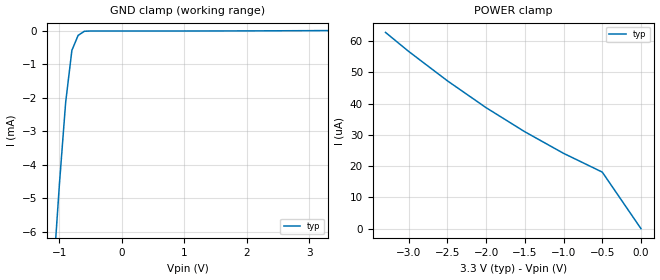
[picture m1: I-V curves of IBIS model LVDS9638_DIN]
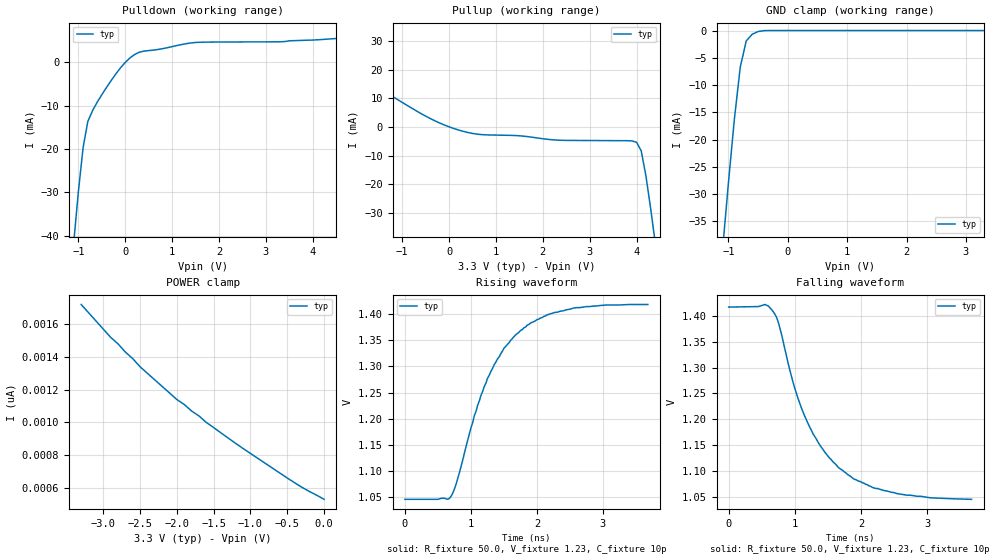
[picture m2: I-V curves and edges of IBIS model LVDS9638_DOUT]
|   Texas Instruments Incorporated
|   Data Transmissions Products
|   IBIS Model for SN65LVDS9638
|   8D SOIC Package
[IBIS Ver]   2.1
[Comment char]   |_char
[File name]   lvds9638.ibs
[File Rev]   2.0
[Date]   27May98
[Source]   File originated at Texas Instruments Incorporated.
   Data Transmission Products Group. All data based on
   Bench Measurements.
[Notes]   Model revved in Nov02 to fix common-mode bug  -TMF-
[Disclaimer]
(C) Copyright Texas Instruments Incorporated 1997
   All rights reserved
  Texas Instruments Incorporated hereby grants the user of this IBIS
model a non-exclusive, nontransferable license to use this IBIS model
under the following terms.  Before using this IBIS model, the user
should read this license.  If the user does not accept these terms,
the IBIS model should be returned to Texas Instruments within 30 days.
  The user is granted this license only to use the IBIS model and
is not granted rights to sell, load, rent, lease or license the IBIS
model in whole or in part, or in modified form to anyone other than
user.  User may modify the IBIS model to suit its specific applications
but rights to derivative works and such modifications shall belong to
Texas Instruments.
  This IBIS model is provided on an "AS IS" basis and Texas Instruments
makes absolutely no warranty with respect to the information contained
herein.  TEXAS INSTRUMENTS DISCLAIMS AND CUSTOMER WAIVES ALL WARRANTIES,
EXPRESS OR IMPLIED, INCLUDING WARRANTIES OF MERCHANTABILITY OR FITNESS
FOR A PARTICULAR PURPOSE. The entire risk as to quality and performance
is with the Customer. ACCORDINGLY, IN NO EVENT SHALL THE COMPANY BE LIABLE
FOR ANY DAMAGES, WHETHER IN CONTRACT OR TORT,INCLUDING ANY LOST PROFITS
OR OTHER INCIDENTAL, CONSEQUENTIAL, EXEMPLARY, OR PUNITIVE DAMAGES ARISING
OUT OF THE USE OR APPLICATION OF THE IBIS model provided in this package.
Further, Texas Instruments reserves the right to discontinue or make changes
without notice to any product herein to improve reliability, function, or
design. Texas Instruments does not convey any license under patent rights
or any other intellectual property rights, including those of third parties.
Contact Texas Instruments at ATTN:DATA TRANSMISSIONS
[Copyright]   Copyright 1997, Texas Instruments, All Rights Reserved
[Component]   SN65LVDS9638D
[Manufacturer]  Texas Instruments Incorporated
[Package]
|   typ   min   max
R_pkg   0.036   0.033   0.039
L_pkg   3.340nH   2.445nH   4.233nH
C_pkg   0.470pF   0.308pF   0.631pF
[Pin]   signal_name   model_name   R_pin   L_pin   C_pin
1   VCC   POWER   0.034   4.233n   0.630p
2   1A   LVDS9638_DIN   0.038   2.445n   0.309p
3   2A   LVDS9638_DIN   0.039   2.448n   0.309p
4   GND   GND   0.033   4.231n   0.631p
5   2Z   LVDS9638_DOUT   0.033   4.230n   0.630p
6   2Y   LVDS9638_DOUT   0.039   2.450n   0.308p
7   1Z   LVDS9638_DOUT   0.039   2.448n   0.309p
8   1Y   LVDS9638_DOUT   0.033   4.231n   0.630p
[Diff_pin]   inv_pin   vdiff   tdelay_typ   tdelay_min   tdelay_max
| The 'xY' pin is Diff_pin and the 'xZ' pin is the inv_pin
6   5   NA   0 0 0
8   7   NA   0 0 0
| Models and submodels in the file (2): LVDS9638_DIN (Input), LVDS9638_DOUT (3-state)
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|   Driver Input  MODEL
[Model]   LVDS9638_DIN
Model_type   Input
|Signals   1A,2A
Vinh = 2.0
Vinl = 0.8
|   typ   min   max
C_comp   1.0pF   NA   NA
|   typ   min   max
[Temperature Range]   25.0   NA   NA
[Voltage range]   3.3V   3.0V   3.6V
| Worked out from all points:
|   GND clamp passes 1 mA (typ) near -0.83 V on its own axis
[GND_clamp]
|   Voltage   I(typ)   I(min)   I(max)
-3.3V     -81mA      NA         NA
-1.1V     -7.36mA    NA         NA
-1V       -4.59mA    NA         NA
-900mV    -2.14mA    NA         NA
-800mV    -579uA     NA         NA
-700mV    -131uA     NA         NA
-600mV    -7.97uA    NA         NA
3.3V      12.9uA     NA         NA
[Power_clamp]
| Note that the[POWER_clamp]voltage table is referenced to Vcc
| and is calculated using Vtable=Vcc - Vmeasured.
|   Voltage   I(typ)   I(min)   I(max)
-3.3V     62.8uA     NA         NA
-3V       56.7uA     NA         NA
-2.5V     47.3uA     NA         NA
-2V       38.7uA     NA         NA
-1.5V     31uA       NA         NA
-1V       24.1uA     NA         NA
-500mV    18.1uA     NA         NA
0V        0A         NA         NA
|   Driver Output  MODEL
[Model]   LVDS9638_DOUT
Model_type   3-state
| Signals   1Y,1Z,2Y,2Z
Vmeas = 1.2V   |Reference voltage for timing measurements
Cref = 10pF   |Timing specification test load capacitance value
Rref = 50   |Note: 50 Ohm load; single ended configuration
Vref = 1.23V   |Timing specification test load voltage
| variable   typ   min   max
C_comp   1.0pF   NA   NA
|   typ   min   max
[Temperature Range]   25.0   NA   NA
[Voltage range]   3.3V   3.0V   3.6V
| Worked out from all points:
|   slope of the pulldown table from 0 to 0.495 V, typ, clamps not added: 182 ohm
|   slope of the pullup table from 0 to 0.495 V, typ, clamps not added: 216 ohm
|   GND clamp passes 1 mA (typ) near -0.63 V on its own axis
|   rising waveform, R_fixture 50.0, V_fixture 1.23, C_fixture 10p: 20-80 % time 692ps typ, NA min, NA max; typ from 1.04 V to 1.42 V
|   falling waveform, R_fixture 50.0, V_fixture 1.23, C_fixture 10p: 20-80 % time 728ps typ, NA min, NA max; typ from 1.42 V to 1.04 V
[Pulldown]
|   Voltage   I(typ)   I(min)   I(max)
-3.3V     -343mA     NA         NA
-1.1V     -41.6mA    NA         NA
-1V       -29.8mA    NA         NA
-900mV    -19.7mA    NA         NA
-800mV    -13.7mA    NA         NA
-600mV    -9.24mA    NA         NA
-200mV    -2.67mA    NA         NA
100mV     992uA      NA         NA
300mV     2.32mA     NA         NA
1.5V      4.56mA     NA         NA
4V        5.12mA     NA         NA
6.6V      7.6mA      NA         NA
[Pullup]
|   Voltage   I(typ)   I(min)   I(max)
| Note that the[Pullup]voltage table is referenced to Vcc
| and is calculated using Vtable=Vcc - Vmeasured.
-3.3V     35mA       NA         NA
-1.2V     10.6mA     NA         NA
-500mV    3.81mA     NA         NA
100mV     -516uA     NA         NA
700mV     -2.67mA    NA         NA
2.3V      -4.58mA    NA         NA
4V        -5.33mA    NA         NA
4.1V      -8.38mA    NA         NA
4.2V      -17.1mA    NA         NA
4.3V      -28.4mA    NA         NA
4.4V      -40.7mA    NA         NA
6.6V      -343mA     NA         NA
[GND_clamp]
|   Voltage   I(typ)   I(min)   I(max)
| Outputs in High Impedance (off)
-3.3V     -343mA     NA         NA
-1.1V     -40.4mA    NA         NA
-1V       -28mA      NA         NA
-900mV    -16.3mA    NA         NA
-800mV    -6.69mA    NA         NA
-700mV    -1.92mA    NA         NA
-600mV    -693uA     NA         NA
-500mV    -186uA     NA         NA
-300mV    -1.48uA    NA         NA
3.3V      531pA      NA         NA
[POWER_clamp]
|   Voltage   I(typ)   I(min)   I(max)
| Note that the [POWER_clamp] voltage table is referenced to Vcc
| and is calculated using Vtable = Vcc - Vmeasured.
| Outputs in Tri-state.
-3.3V     1.72nA     NA         NA
-2.9V     1.52nA     NA         NA
-2.8V     1.48nA     NA         NA
-2.5V     1.34nA     NA         NA
-2V       1.14nA     NA         NA
-1.9V     1.11nA     NA         NA
-1.6V     1nA        NA         NA
-1.1V     841pA      NA         NA
-400mV    632pA      NA         NA
0V        531pA      NA         NA
[Ramp]
| Note: Ramp rate measured on single-ended Driver Output.
|   typ   min   max
dV/dt_r   0.224/684ps   NA   NA
dV/dt_f   0.223/732ps   NA   NA
R_load = 50ohm | Note: These are single ended driver measurements
|   with 100ohm line-to-line termination and 4.5pF
|   line-to-ground capacitive load
[Rising Waveform]
R_fixture = 50.0
V_fixture = 1.23
C_fixture = 10p
L_fixture = 0n
|   V(typ)   V(min)   V(max)
0s        1.045V     NA         NA
700ps     1.051V     NA         NA
775ps     1.074V     NA         NA
1.05ns    1.205V     NA         NA
1.25ns    1.277V     NA         NA
1.5ns     1.335V     NA         NA
1.75ns    1.369V     NA         NA
2.15ns    1.399V     NA         NA
2.55ns    1.412V     NA         NA
3.68ns    1.419V     NA         NA
[Falling Waveform]
R_fixture = 50.0
V_fixture = 1.23
C_fixture = 10p
L_fixture = 0n
|   V(typ)   V(min)   V(max)
0s        1.417V     NA         NA
550ps     1.422V     NA         NA
675ps     1.408V     NA         NA
750ps     1.388V     NA         NA
975ps     1.271V     NA         NA
1.15ns    1.206V     NA         NA
1.4ns     1.146V     NA         NA
1.675ns   1.105V     NA         NA
2.45ns    1.059V     NA         NA
3.675ns   1.045V     NA         NA
